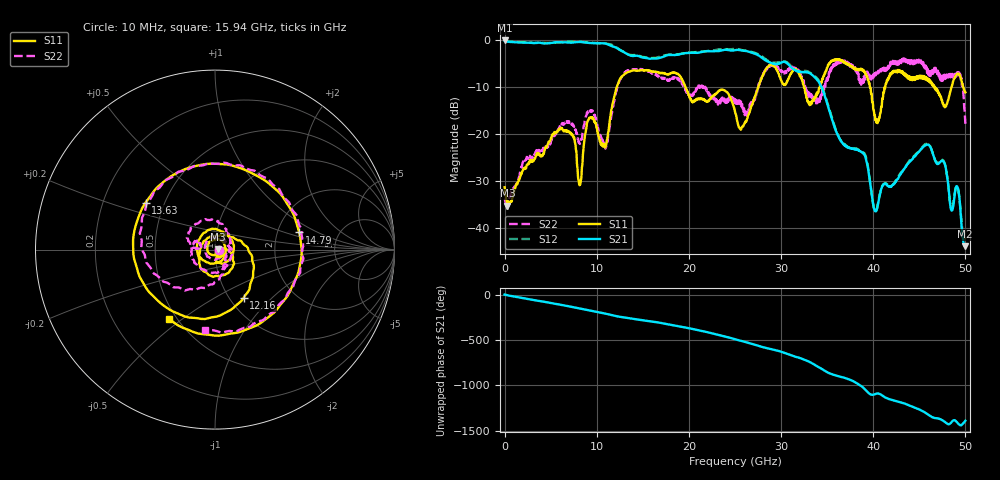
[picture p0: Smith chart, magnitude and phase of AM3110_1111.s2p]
# Hz S DB R 50.0
!freq dBS11 angS11 dBS21 angS21 dBS12 angS12 dBS22 angS22
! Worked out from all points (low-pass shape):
!   1601 points, 10 MHz to 50 GHz, reference 50 ohm
!   highest |S21| = -0.01 dB at 10 MHz (marker M1); lowest = -43.9 dB at 49.91 GHz (marker M2)
!   |S21| within 3 dB of the highest: start of sweep to 13.38 GHz; 18.87 GHz to 27.36 GHz (8.485 GHz wide, 36.7 % of centre)
!   lowest |S11| = -35.3 dB at 322.4 MHz (marker M3), VSWR 1.03, Z = 51.7 + j0.184 ohm
!   |S11| at or under -10 dB: start of sweep to 12.18 GHz; 19.65 GHz to 27.53 GHz (7.886 GHz wide, 33.4 % of centre); 46.72 GHz to 48.49 GHz (1.772 GHz wide, 3.72 % of centre)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
!   |S22| runs from -36.2 to -3.9 dB; largest |S21 - S12| = 0.032
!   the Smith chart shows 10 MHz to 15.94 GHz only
!   S11 on the Smith chart (normalised r, x): 10 MHz: 1.04, -0.04; 12.16 GHz: 1.16, -0.69; 13.63 GHz: 0.39, +0.26; 14.79 GHz: 2.65, +0.66; 15.94 GHz: 0.46, -0.45
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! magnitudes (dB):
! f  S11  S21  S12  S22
! 10 MHz  -31.4  0.0  -0.1  -33.8
! 322.4 MHz  -35.3  -0.3  -0.2  -35.7
! 6.009 GHz  -18.7  -0.4  -0.4  -18.2
! 8.352 GHz  -28.8  -0.4  -0.3  -21.0
! 9.196 GHz  -16.5  -0.5  -0.5  -14.8
! 10.95 GHz  -22.6  -0.7  -0.7  -23.1
! 12.16 GHz  -10.1  -1.6  -1.5  -10.7
! 13.63 GHz  -6.6  -3.2  -3.1  -6.4
! 14.79 GHz  -6.4  -3.5  -3.4  -6.3
! 15.94 GHz  -6.7  -3.9  -3.8  -6.9
! 16.69 GHz  -6.8  -3.8  -3.6  -7.7
! 25 GHz  -15.2  -2.1  -1.8  -12.8
! 28.91 GHz  -5.2  -4.8  -4.7  -5.2
! 33.35 GHz  -13.5  -7.3  -7.2  -12.6
! 36.32 GHz  -4.0  -20.9  -20.9  -4.4
! 39.06 GHz  -6.8  -24.4  -24.1  -8.4
! 40.19 GHz  -16.2  -36.3  -36.4  -7.0
! 41.69 GHz  -7.9  -31.1  -30.8  -5.9
! 46.03 GHz  -8.6  -22.3  -22.1  -6.4
! 49.16 GHz  -7.1  -31.4  -31.5  -7.5
! 49.91 GHz  -10.9  -43.9  -42.4  -14.9
! 50 GHz  -11.1  -43.5  -42.1  -17.8
